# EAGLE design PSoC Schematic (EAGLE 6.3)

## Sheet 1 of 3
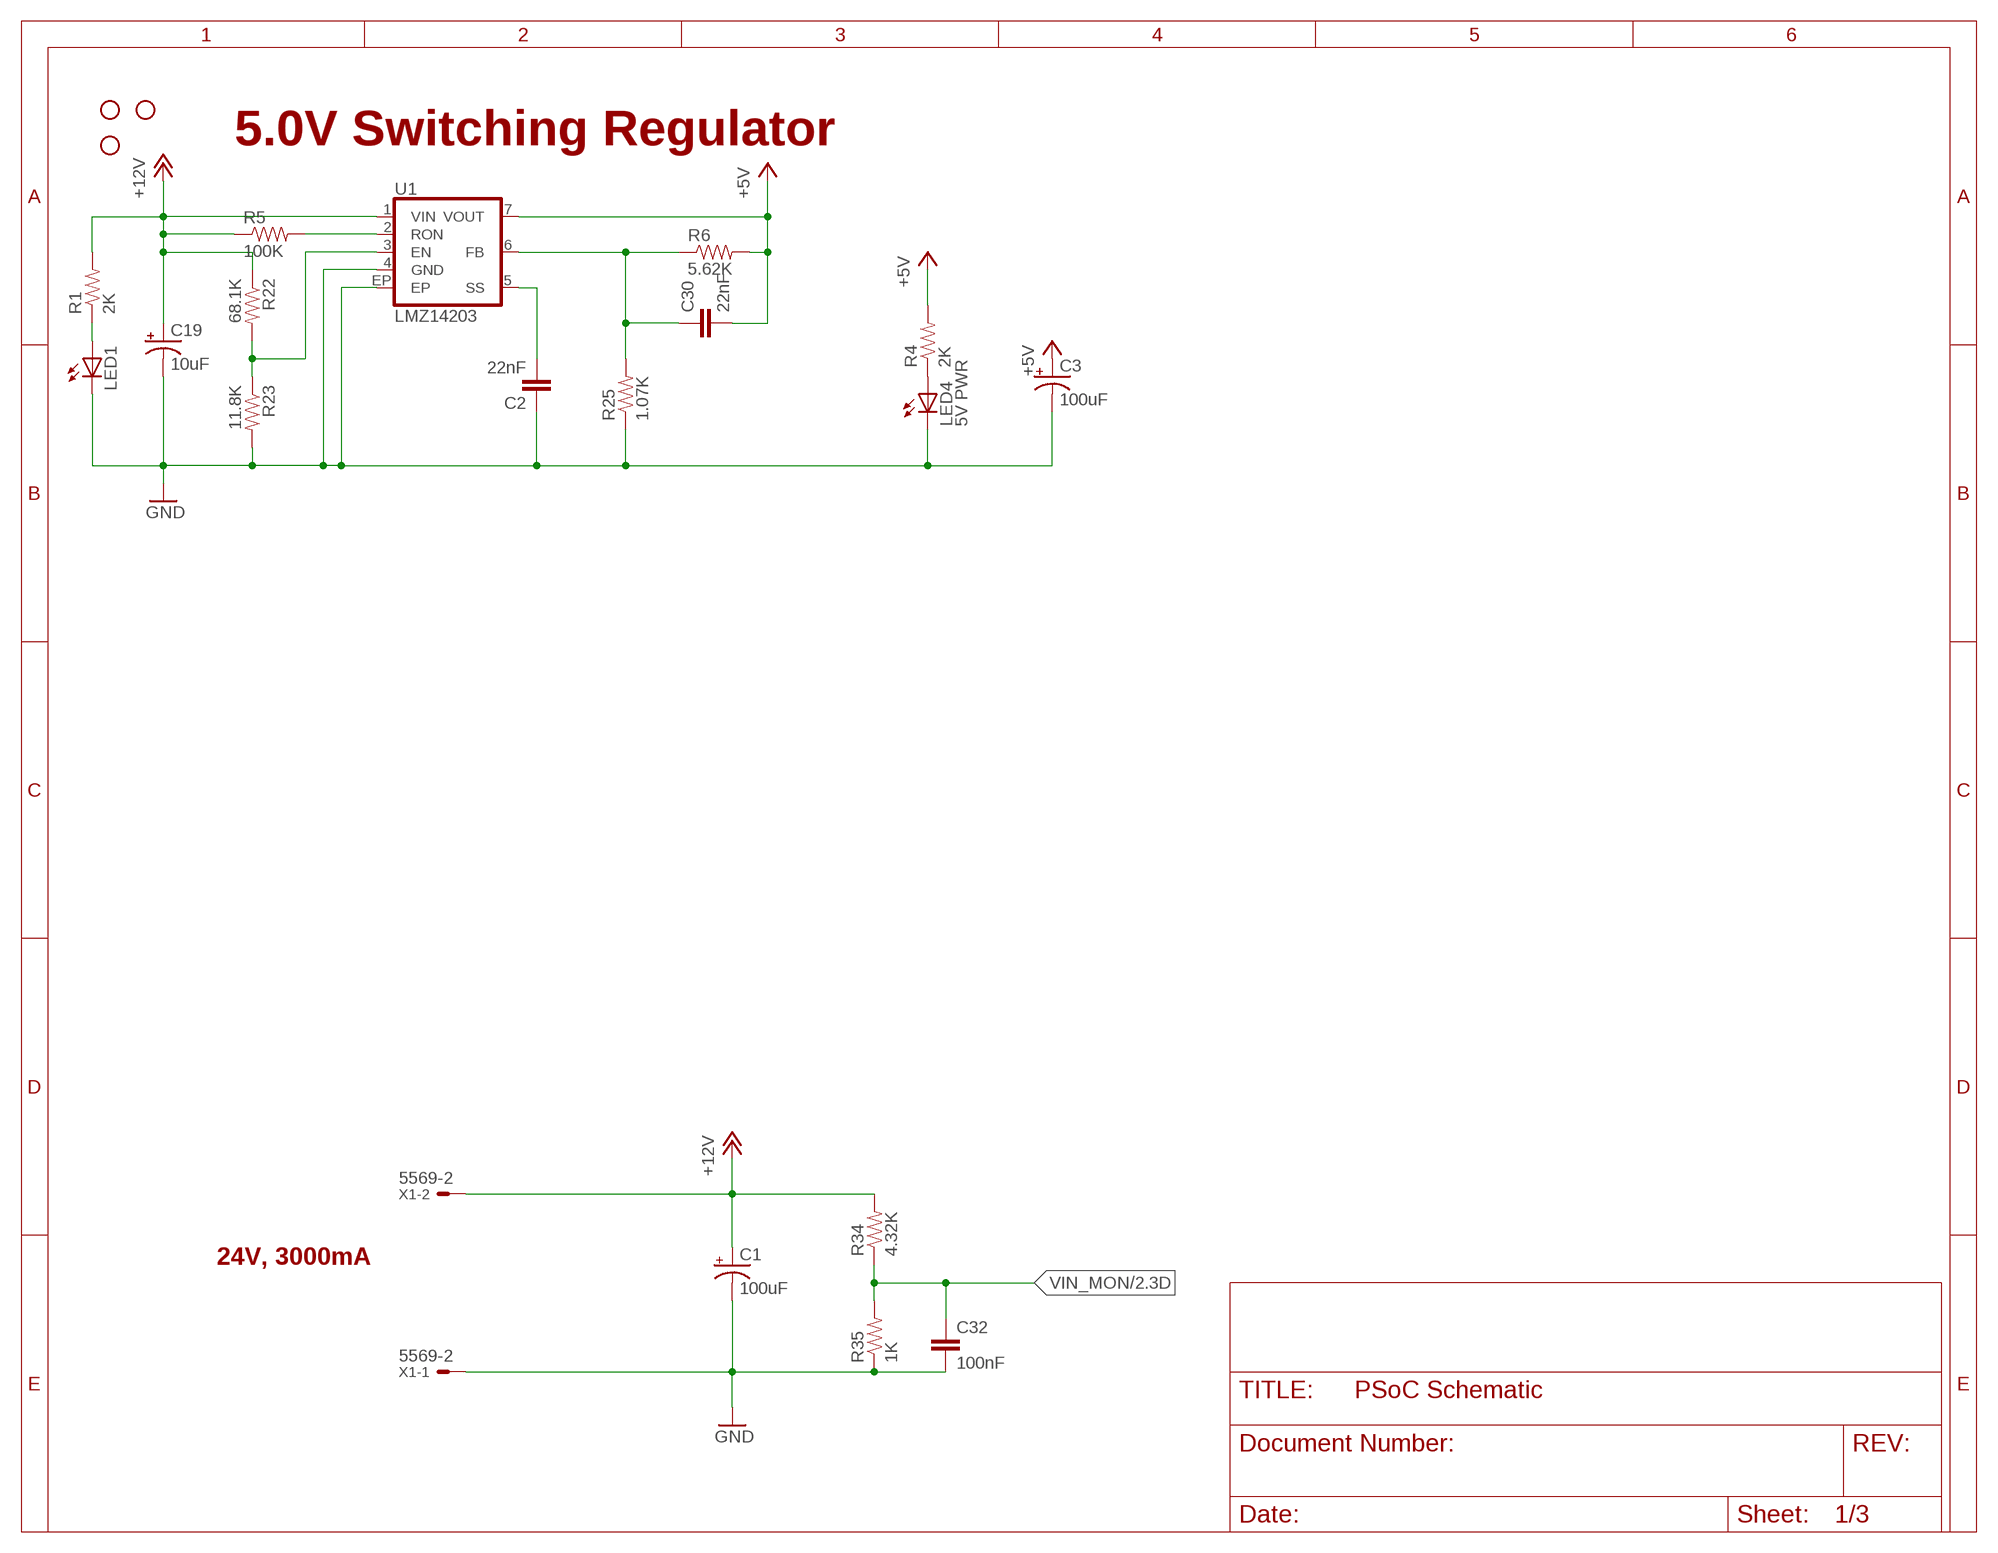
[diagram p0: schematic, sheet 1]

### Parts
C1  100uF  CAP_POLE  [PANASONIC_E]
C2  22nF  22UF-6.3V-20%(0805)  [0805]
C3  100uF  CAP_POLE  [PANASONIC_E]
C19  10uF  CAP_POL3528  [EIA3528]
C30  22nF  CAP1206  [1206]
C32  100nF  CAP1206  [1206]
JP6  SPARKFUN_STAND-OFF  [SPARKFUN_STAND-OFF]
JP7  SPARKFUN_STAND-OFF  [SPARKFUN_STAND-OFF]
JP8  SPARKFUN_STAND-OFF  [SPARKFUN_STAND-OFF]
LED1  LED1206  [LED-1206]
LED4  5V PWR  LED1206  [LED-1206]
R1  2K  RESISTOR1206  [1206]
R4  2K  RESISTOR1206  [1206]
R5  100K  RESISTOR0805-RES  [0805]
R6  5.62K  RESISTOR0805-RES  [0805]
R22  68.1K  RESISTOR1206  [1206]
R23  11.8K  RESISTOR1206  [1206]
R25  1.07K  RESISTOR1206  [1206]
R34  4.32K  RESISTOR1206  [1206]
R35  1K  RESISTOR1206  [1206]
U1  LMZ14203  [TO-PMOD-7]
U$2  MUD  [MUD]
X1  5569-2  [5569-2]

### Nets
+5V: C3.+ C30.2 R4.2 R6.2 U1.7(VOUT) ; also sheet 2,3
+12V: C1.+ C19.A(+) R1.2 R5.1 R22.1 R34.2 U1.1(VIN) X1.2 ; also sheet 3
GND: C1.- C2.1 C3.- C19.C(-) C32.2 LED1.C LED4.C R23.2 R25.1 R35.1 U1.4(GND) U1.EP X1.1 ; also sheet 2,3
N$2: LED4.A R4.1
N$3: LED1.A R1.1
N$60: R5.2 U1.2(RON)
N$62: R22.2 R23.1 U1.3(EN)
N$66: C2.2 U1.5(SS)
N$67: C30.1 R6.1 R25.2 U1.6(FB)
VIN_MON: C32.1 R34.1 R35.2 ; also sheet 2

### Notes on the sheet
- 5.0V Switching Regulator
- 24V, 3000mA

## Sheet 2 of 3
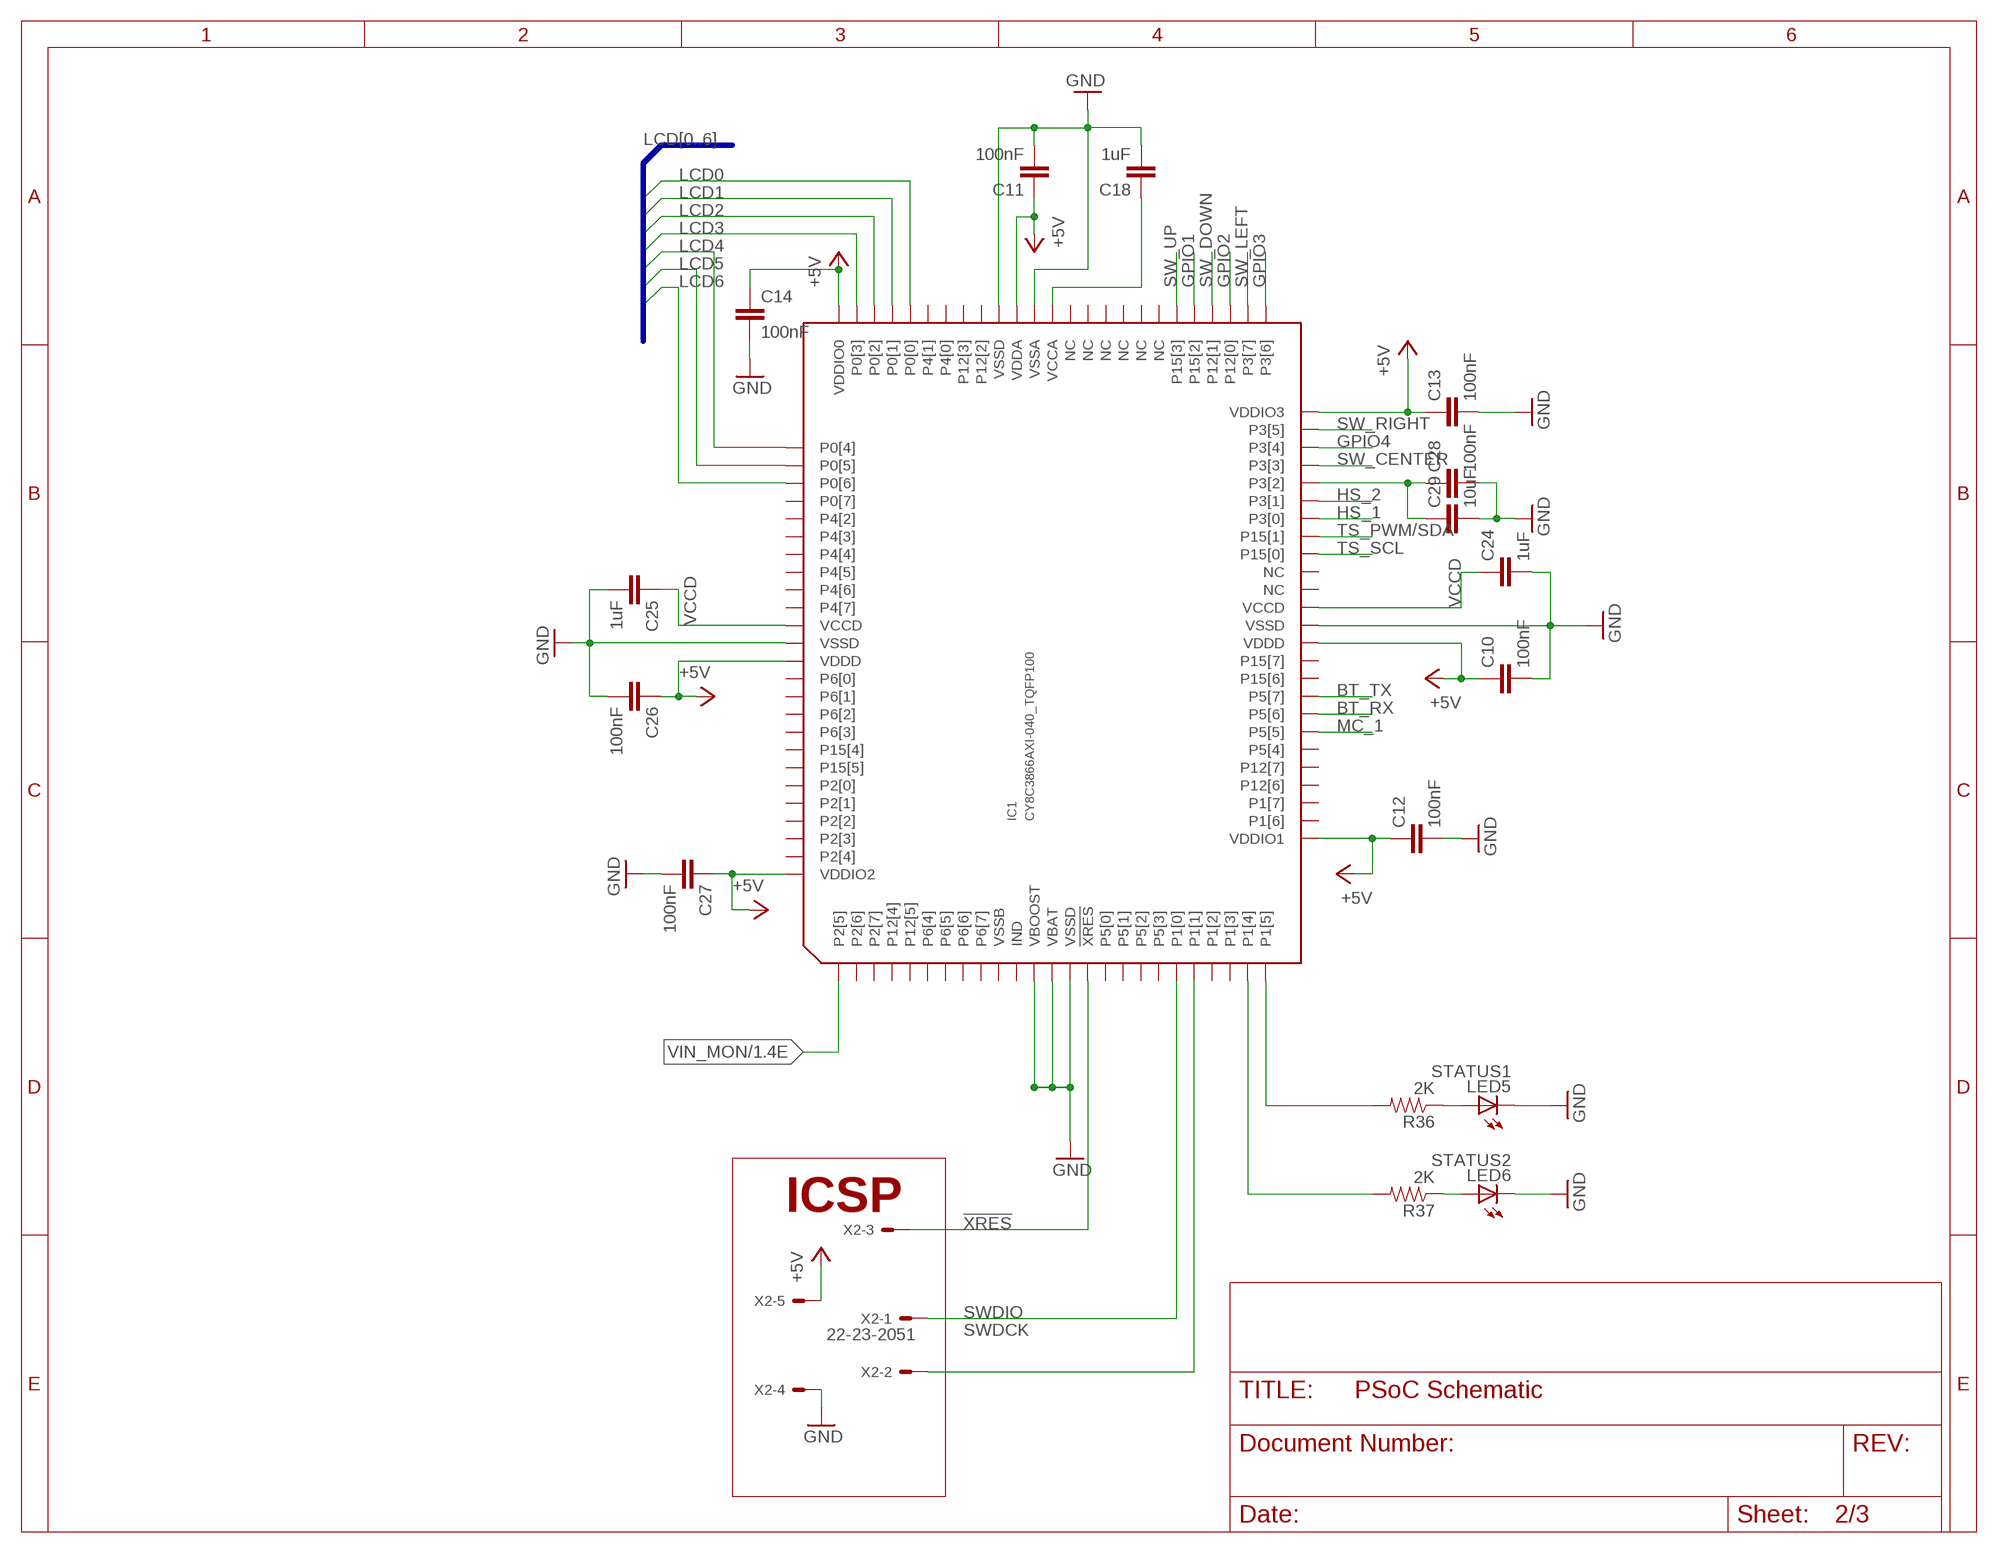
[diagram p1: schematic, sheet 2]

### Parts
C10  100nF  CAP1206  [1206]
C11  100nF  CAP1206  [1206]
C12  100nF  CAP1206  [1206]
C13  100nF  CAP1206  [1206]
C14  100nF  CAP1206  [1206]
C18  1uF  CAP1206  [1206]
C24  1uF  CAP1206  [1206]
C25  1uF  CAP1206  [1206]
C26  100nF  CAP1206  [1206]
C27  100nF  CAP1206  [1206]
C28  100nF  CAP1206  [1206]
C29  10uF  CAP1206  [1206]
IC1  CY8C3866AXI-040_TQFP100  [TQFP100]
LED5  STATUS1  LED1206  [LED-1206]
LED6  STATUS2  LED1206  [LED-1206]
R36  2K  RESISTOR1206  [1206]
R37  2K  RESISTOR1206  [1206]
X2  22-23-2051  [22-23-2051]

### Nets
!XRES: IC1.15(!XRES) X2.3
+5V: C10.1 C11.1 C12.1 C13.1 C14.1 C26.1 C27.1 IC1.26(VDDIO1) IC1.37(VDDD) IC1.50(VDDIO3) IC1.65(VDDA) IC1.75(VDDIO0) IC1.88(VDDD) IC1.100(VDDIO2) X2.5 ; also sheet 1,3
BT_RX: IC1.33(P5[6]) ; also sheet 3
BT_TX: IC1.34(P5[7]) ; also sheet 3
GND: C10.2 C11.2 C12.2 C13.2 C14.2 C18.2 C24.2 C25.2 C26.2 C27.2 C28.2 C29.2 IC1.12(VBOOST) IC1.13(VBAT) IC1.14(VSSD) IC1.38(VSSD) IC1.64(VSSA) IC1.66(VSSD) IC1.87(VSSD) LED5.C LED6.C X2.4 ; also sheet 1,3
GPIO1: IC1.55(P15[2]) ; also sheet 3
GPIO2: IC1.53(P12[0]) ; also sheet 3
GPIO3: IC1.51(P3[6]) ; also sheet 3
GPIO4: IC1.48(P3[4]) ; also sheet 3
HS_1: IC1.44(P3[0]) ; also sheet 3
HS_2: IC1.45(P3[1]) ; also sheet 3
LCD0: IC1.71(P0[0]) ; also sheet 3
LCD1: IC1.72(P0[1]) ; also sheet 3
LCD2: IC1.73(P0[2]) ; also sheet 3
LCD3: IC1.74(P0[3]) ; also sheet 3
LCD4: IC1.76(P0[4]) ; also sheet 3
LCD5: IC1.77(P0[5]) ; also sheet 3
LCD6: IC1.78(P0[6]) ; also sheet 3
MC_1: IC1.32(P5[5]) ; also sheet 3
N$10: LED5.A R36.1
N$20: IC1.25(P1[5]) R36.2
N$26: C18.1 IC1.63(VCCA)
N$28: C28.1 C29.1 IC1.46(P3[2])
N$29: LED6.A R37.1
N$32: IC1.24(P1[4]) R37.2
SW_CENTER: IC1.47(P3[3]) ; also sheet 3
SW_DOWN: IC1.54(P12[1]) ; also sheet 3
SW_LEFT: IC1.52(P3[7]) ; also sheet 3
SW_RIGHT: IC1.49(P3[5]) ; also sheet 3
SW_UP: IC1.56(P15[3]) ; also sheet 3
SWDCK: IC1.21(P1[1]) X2.2
SWDIO: IC1.20(P1[0]) X2.1
TS_PWM/SDA: IC1.43(P15[1]) ; also sheet 3
TS_SCL: IC1.42(P15[0]) ; also sheet 3
VCCD: C24.1 C25.1 IC1.39(VCCD) IC1.86(VCCD)
VIN_MON: IC1.1(P2[5]) ; also sheet 1
Unconnected: IC1.2(P2[6]) IC1.3(P2[7]) IC1.4(P12[4]) IC1.5(P12[5]) IC1.6(P6[4]) IC1.7(P6[5]) IC1.8(P6[6]) IC1.9(P6[7]) IC1.11(IND) IC1.16(P5[0]) IC1.17(P5[1]) IC1.18(P5[2]) IC1.19(P5[3]) IC1.22(P1[2]) IC1.23(P1[3]) IC1.27(P1[6]) IC1.28(P1[7]) IC1.29(P12[6]) IC1.30(P12[7]) IC1.31(P5[4]) IC1.35(P15[6]) IC1.36(P15[7]) IC1.40(NC) IC1.41(NC) IC1.57(NC) IC1.58(NC) IC1.59(NC) IC1.60(NC) IC1.61(NC) IC1.62(NC) IC1.67(P12[2]) IC1.68(P12[3]) IC1.69(P4[0]) IC1.70(P4[1]) IC1.79(P0[7]) IC1.80(P4[2]) IC1.81(P4[3]) IC1.82(P4[4]) IC1.83(P4[5]) IC1.84(P4[6]) IC1.85(P4[7]) IC1.89(P6[0]) IC1.90(P6[1]) IC1.91(P6[2]) IC1.92(P6[3]) IC1.93(P15[4]) IC1.94(P15[5]) IC1.95(P2[0]) IC1.96(P2[1]) IC1.97(P2[2]) IC1.98(P2[3]) IC1.99(P2[4])

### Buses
LCD[0..6]

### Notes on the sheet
- ICSP

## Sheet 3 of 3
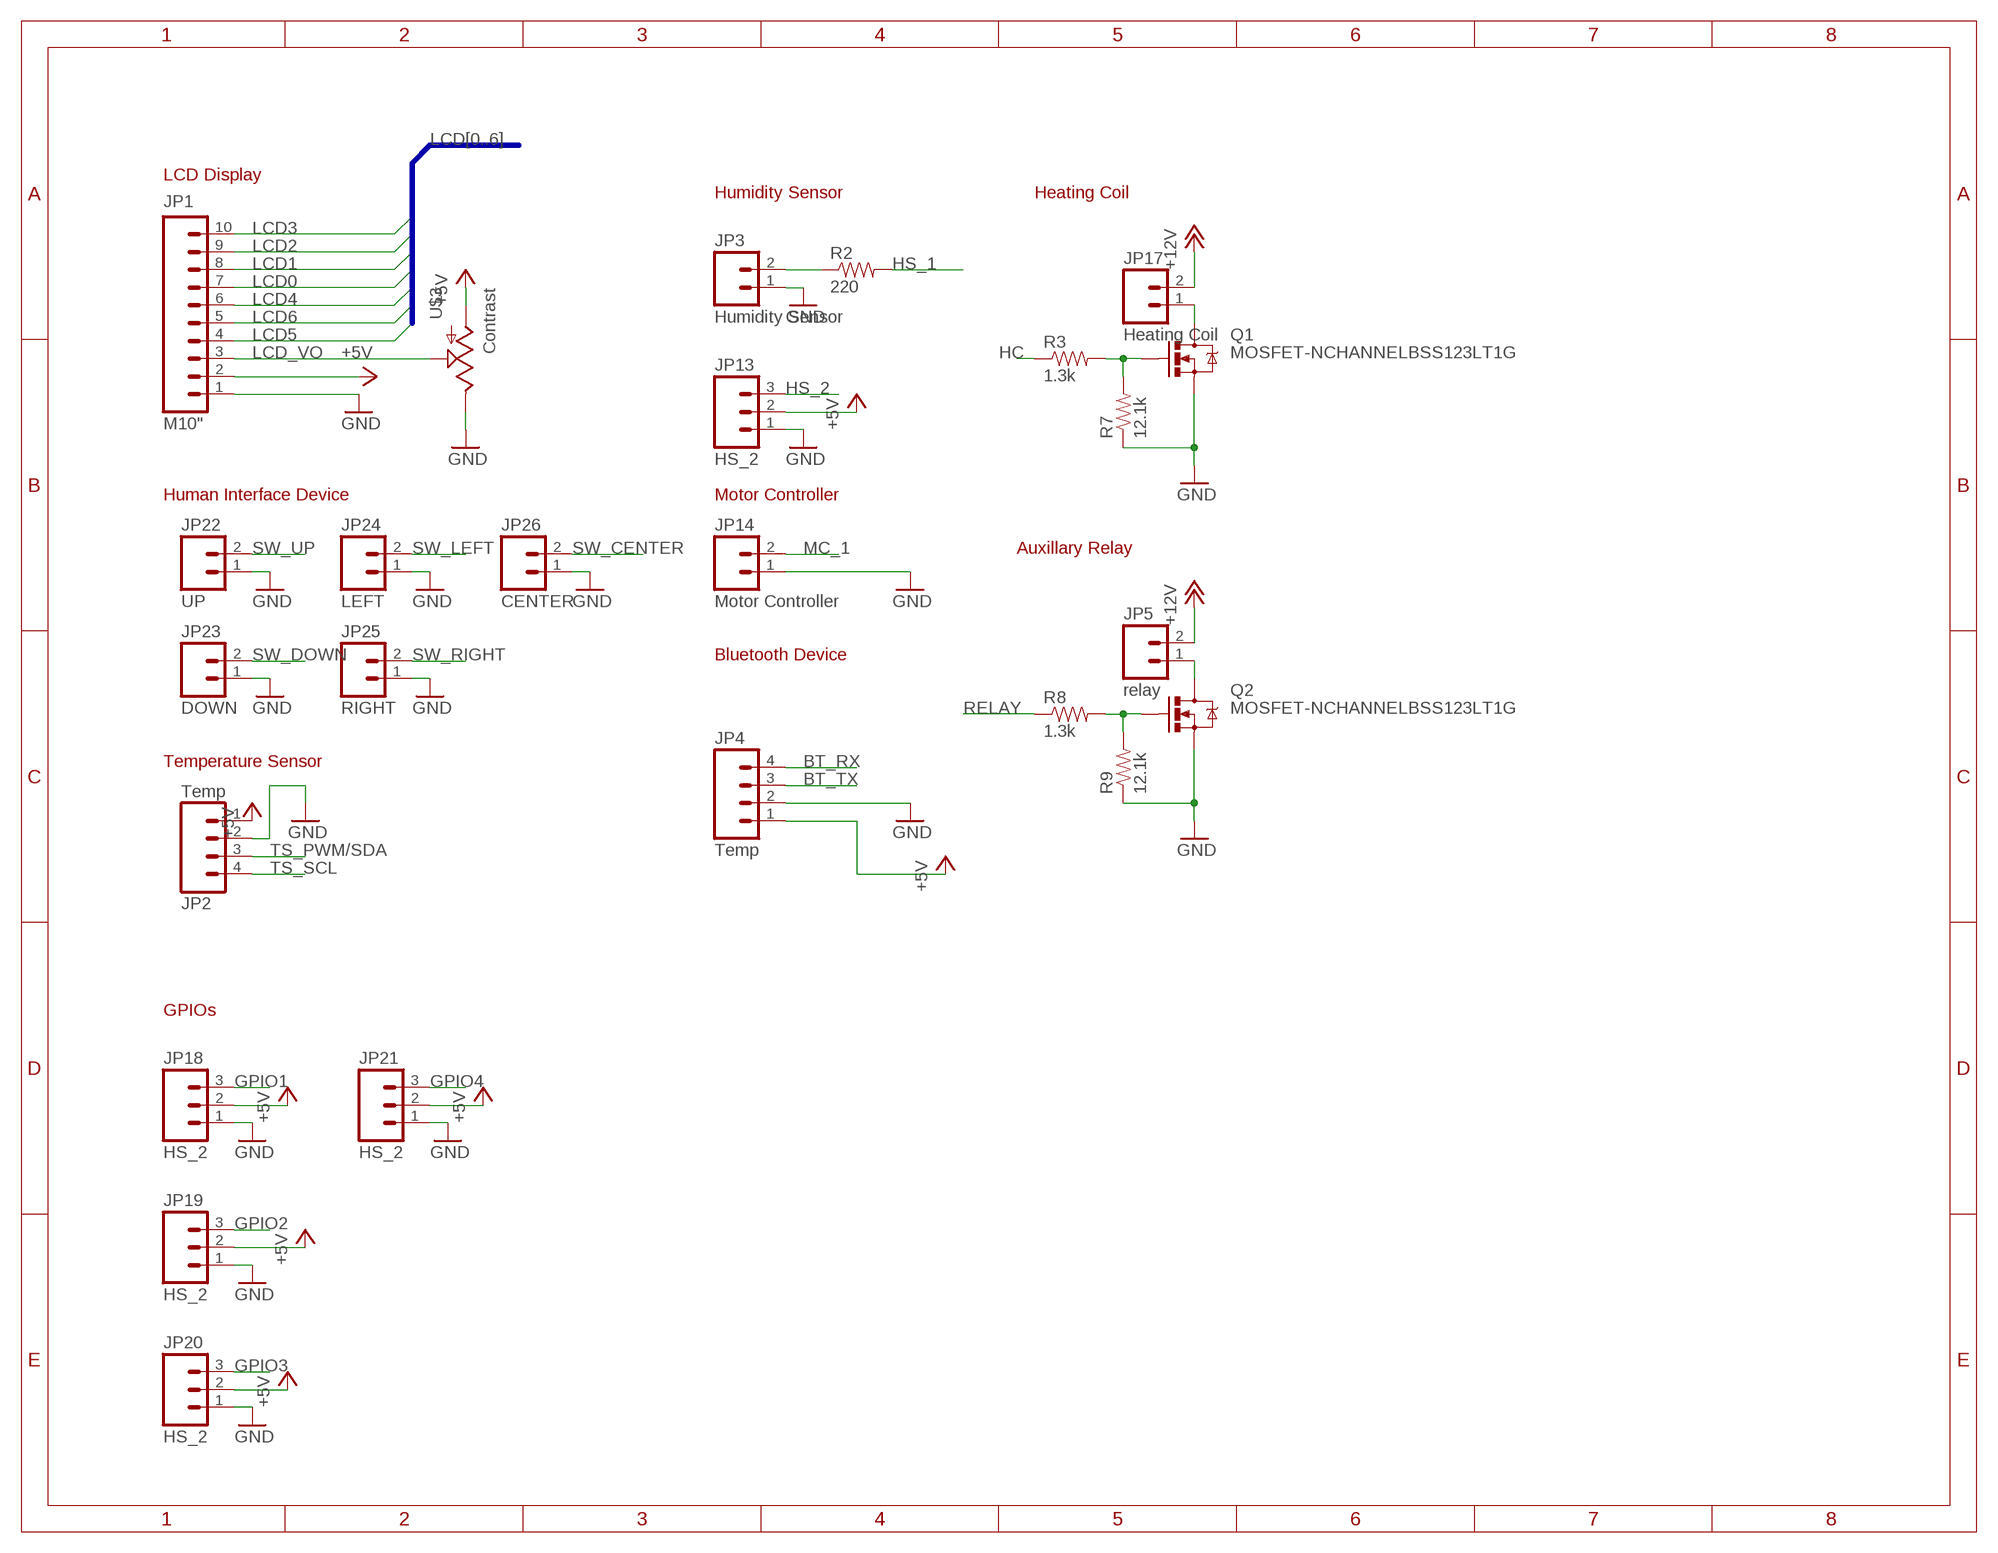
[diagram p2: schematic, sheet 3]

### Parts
JP1  M10"  [1X10]
JP2  Temp  M04POLAR  [MOLEX-1X4]
JP3  Humidity Sensor  M02POLAR  [MOLEX-1X2]
JP4  Temp  M04POLAR  [MOLEX-1X4]
JP5  relay  M02POLAR  [MOLEX-1X2]
JP13  HS_2  M03POLAR  [MOLEX-1X3]
JP14  Motor Controller  M02POLAR  [MOLEX-1X2]
JP17  Heating Coil  M02POLAR  [MOLEX-1X2]
JP18  HS_2  M03POLAR  [MOLEX-1X3]
JP19  HS_2  M03POLAR  [MOLEX-1X3]
JP20  HS_2  M03POLAR  [MOLEX-1X3]
JP21  HS_2  M03POLAR  [MOLEX-1X3]
JP22  UP  M02POLAR  [MOLEX-1X2]
JP23  DOWN  M02POLAR  [MOLEX-1X2]
JP24  LEFT  M02POLAR  [MOLEX-1X2]
JP25  RIGHT  M02POLAR  [MOLEX-1X2]
JP26  CENTER  M02POLAR  [MOLEX-1X2]
Q1  MOSFET-NCHANNELBSS123LT1G  [SOT23]
Q2  MOSFET-NCHANNELBSS123LT1G  [SOT23]
R2  220  220-5%  [0603-RES]
R3  1.3k  RESISTOR1206  [1206]
R7  12.1k  RESISTOR1206  [1206]
R8  1.3k  RESISTOR1206  [1206]
R9  12.1k  RESISTOR1206  [1206]
U$3  Contrast  POT100K_3362U  [3362U]

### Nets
+5V: JP1.2 JP2.1 JP4.1 JP13.2 JP18.2 JP19.2 JP20.2 JP21.2 U$3.P$3(A) ; also sheet 1,2
+12V: JP5.2 JP17.2 ; also sheet 1
BT_RX: JP4.4 ; also sheet 2
BT_TX: JP4.3 ; also sheet 2
GND: JP1.1 JP2.2 JP3.1 JP4.2 JP13.1 JP14.1 JP18.1 JP19.1 JP20.1 JP21.1 JP22.1 JP23.1 JP24.1 JP25.1 JP26.1 Q1.2(S) Q2.2(S) R7.1 R9.1 U$3.P$1(E) ; also sheet 1,2
GPIO1: JP18.3 ; also sheet 2
GPIO2: JP19.3 ; also sheet 2
GPIO3: JP20.3 ; also sheet 2
GPIO4: JP21.3 ; also sheet 2
HC: R3.1
HS_1: R2.2 ; also sheet 2
HS_2: JP13.3 ; also sheet 2
LCD0: JP1.7 ; also sheet 2
LCD1: JP1.8 ; also sheet 2
LCD2: JP1.9 ; also sheet 2
LCD3: JP1.10 ; also sheet 2
LCD4: JP1.6 ; also sheet 2
LCD5: JP1.4 ; also sheet 2
LCD6: JP1.5 ; also sheet 2
LCD_VO: JP1.3 U$3.P$2(S)
MC_1: JP14.2 ; also sheet 2
N$1: JP3.2 R2.1
N$4: Q1.1(G) R3.2 R7.2
N$5: JP17.1 Q1.3(D)
N$7: Q2.1(G) R8.2 R9.2
N$8: JP5.1 Q2.3(D)
RELAY: R8.1
SW_CENTER: JP26.2 ; also sheet 2
SW_DOWN: JP23.2 ; also sheet 2
SW_LEFT: JP24.2 ; also sheet 2
SW_RIGHT: JP25.2 ; also sheet 2
SW_UP: JP22.2 ; also sheet 2
TS_PWM/SDA: JP2.3 ; also sheet 2
TS_SCL: JP2.4 ; also sheet 2

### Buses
LCD[0..6]

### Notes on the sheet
- LCD Display
- Humidity Sensor | Heating Coil
- Human Interface Device | Motor Controller
- Auxillary Relay
- Bluetooth Device
- Temperature Sensor
- GPIOs

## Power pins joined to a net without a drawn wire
VSSB: IC1.10(VSSB)

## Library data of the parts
C1 C3 C19 = SparkFun:CAP_POL: Capacitor Polarized
C2 = SparkFun-Capacitors:22UF-6.3V-20%(0805): Ceramic; PROD_ID: CAP-08402; VALUE: 22uF
C10-C14 C18 C24-C30 C32 = SparkFun:CAP: Capacitor
IC1 = cypresspsoc_0.30:CY8C3866AXI-040
JP1 = SparkFun-Connectors:M10: Header 10 Standard 10-pin 0.1" header. Use with straight break away headers (SKU : PRT-00116), right angle break away headers (PRT-00553), swiss pins (PRT-00743), machine pins (PRT-00117), and female headers (PRT-00115).
JP2 JP4 = SparkFun-Connectors:M04: Header 4 Standard 4-pin 0.1" header. Use with straight break away headers (SKU : PRT-00116), right angle break away headers (PRT-00553), swiss pins (PRT-00743), machine pins (PRT-00117), and female headers (PRT-00115). Molex polarized connector foot print use with SKU : PRT-08231 with associated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
JP3 JP5 JP14 JP17 JP22-JP26 = SparkFun-Connectors:M02: Header 2
JP6-JP8 = IOIO-OTG-v20brandon2-14-13:SPARKFUN_STAND-OFF: Stand Off
JP13 JP18-JP21 = SparkFun-Connectors:M03: Header 3 Standard 3-pin 0.1" header. Use with straight break away headers (SKU : PRT-00116), right angle break away headers (PRT-00553), swiss pins (PRT-00743), machine pins (PRT-00117), and female headers (PRT-00115). Molex polarized connector foot print use with SKU : PRT-08232 with associated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
LED1 LED4-LED6 = SparkFun:LED: LEDs
Q1 Q2 = SparkFun-DiscreteSemi:MOSFET-NCHANNEL: Common NMOSFET Parts MFG P/NStore IDProd ID FDD8780TRANS-09984 SI7820DNTRANS-11055 FDS6630AIC-08089 2N7002PWTRANS-11151 FQP30N06L COM-10213TRANS-10060 BSS123LT1GTRANS-08345 BSS138TRANS-00830 BS170 2N7000; PROD_ID: TRANS-08345
R1 R4 R22 R23 R25 R34-R37 = SparkFun:RESISTOR: Resistor
R2 = SparkFun-Resistors:220-5%: 220-ohm SMT; PROD_ID: RES-07866
R3 R5-R9 = SparkFun-Passives:RESISTOR: Resistor
U1 = SparkFun:LMZ14203: LMZ14203 3A, Simple Switcher Power Module with 42V Maximum Input
U$2 = logo:MUD
U$3 = SparkFun-Electromechanical:POT
X1 = molex:5569-2: Mini FIT connector 2 pol; OC_FARNELL: 1822072; OC_NEWARK: unknown
X2 = con-molex:22-23-2051: .100" (2.54mm) Center Header - 5 Pin; MF: MOLEX; MPN: 22-23-2051; OC_FARNELL: 1462952; OC_NEWARK: 38C9178

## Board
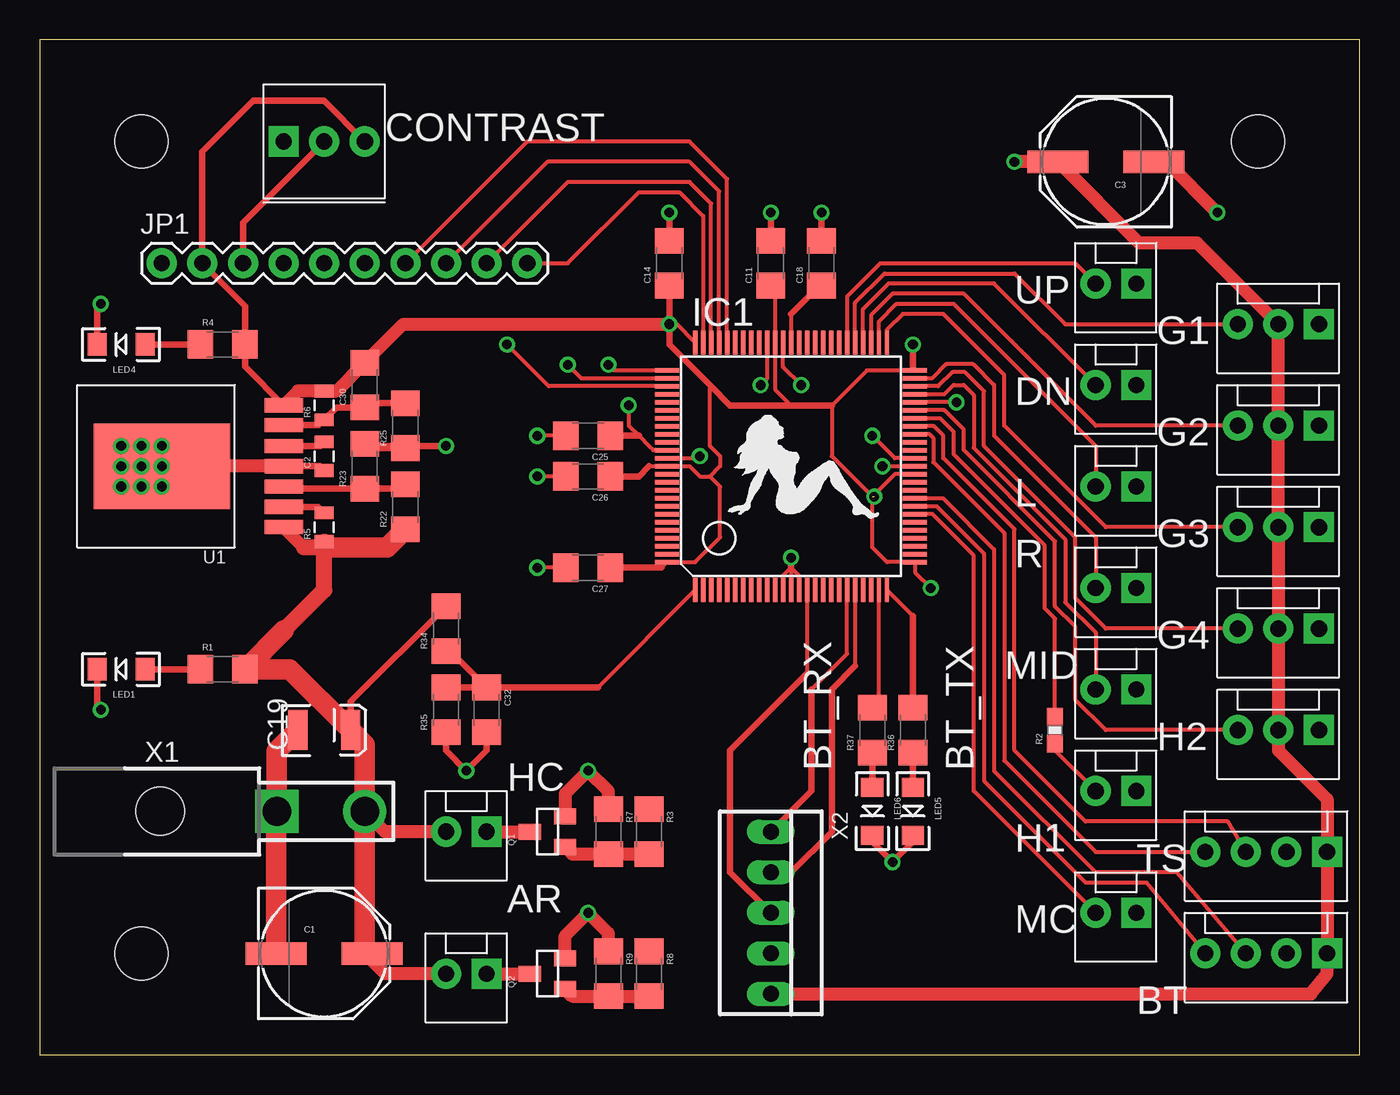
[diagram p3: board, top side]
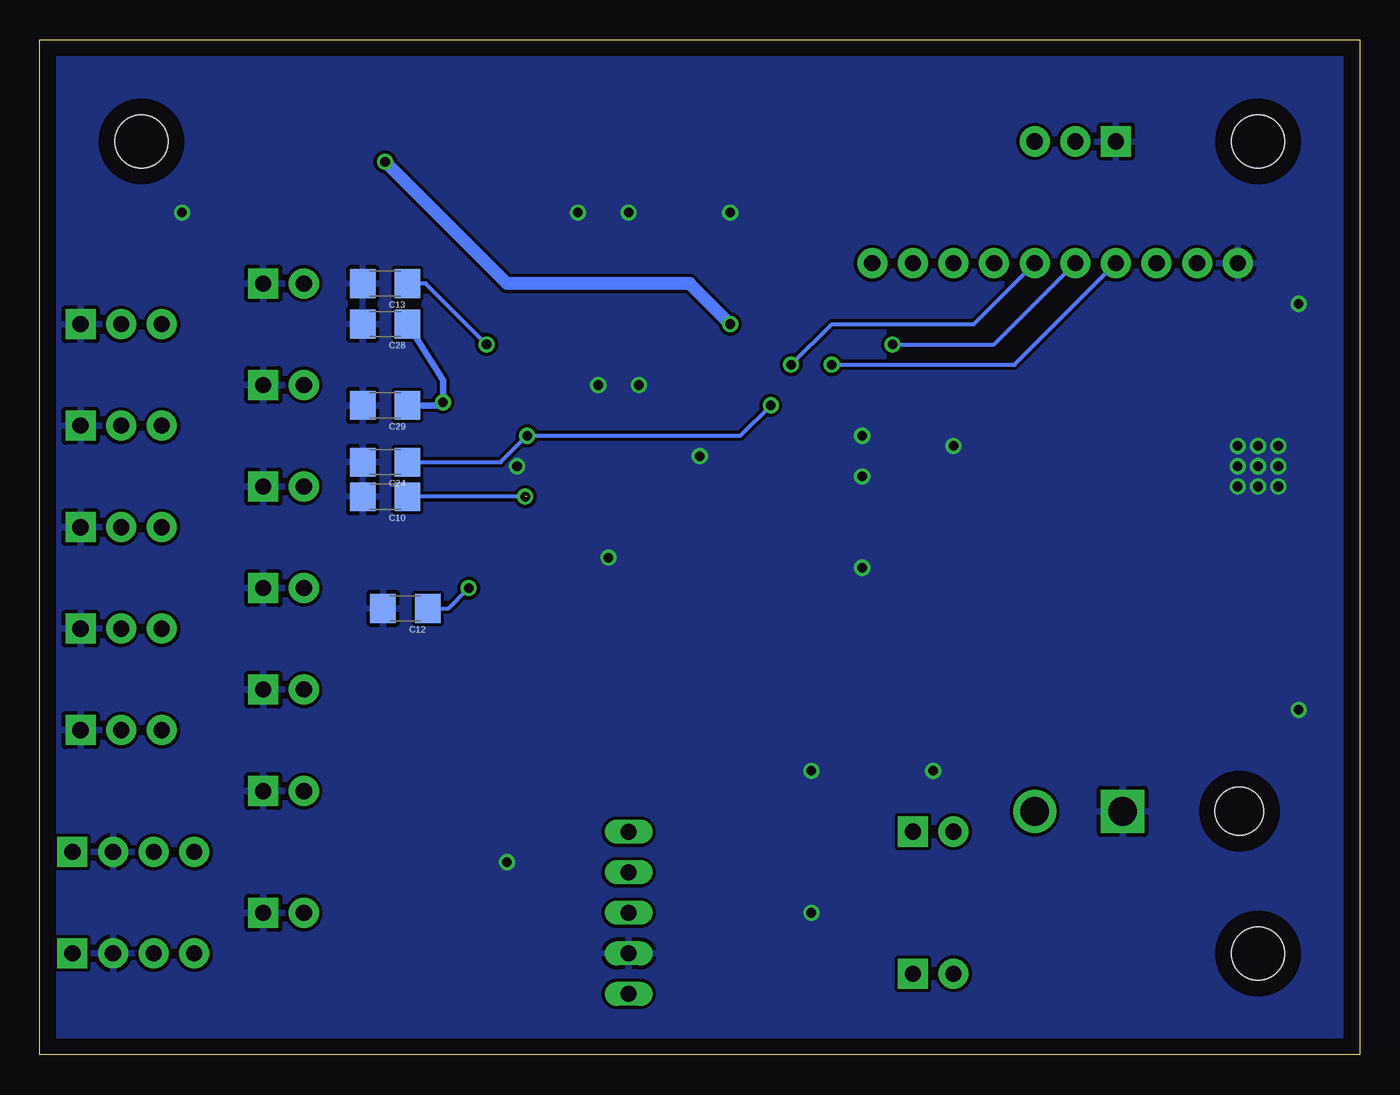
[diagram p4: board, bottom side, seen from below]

Size 82.55 x 63.5 mm. Coordinates in mm from the lower left corner, seen from the top.
Outline: 0,0 82.55,0 82.55,63.5 0,63.5 0,0
Copper layers (1*16): Top 0.035mm / dielectric 1.5mm / Bottom 0.035mm
Design rules "default": minimum track width 10mil, minimum drill 24mil, track to track 8mil, track to pad 8mil, pad to pad 8mil, via to via 8mil, smd to smd 8mil, copper to edge 40mil, drill to drill 8mil, minimum pad ring 10mil, minimum via ring 8mil, stop-mask expansion 4mil, vias tented up to drill 0mil, thermal gap 10mil

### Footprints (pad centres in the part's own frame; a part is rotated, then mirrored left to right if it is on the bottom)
PANASONIC_E = smd 3.8 x 1.4: + 3,0; - -3,0
0805 = smd 0.8 x 1.2: 1 -0.9,0; 2 0.9,0
1206 = smd 1.6 x 1.8: 1 -1.4,0; 2 1.4,0
EIA3528 = smd 1.2 x 2.5: A 1.65,0; C -1.65,0
TQFP100 = smd 0.27 x 1.5: 1 -6,-7.75; 2 -5.5,-7.75; 3 -5,-7.75; 4 -4.5,-7.75; 5 -4,-7.75; 6 -3.5,-7.75; 7 -3,-7.75; 8 -2.5,-7.75; 9 -2,-7.75; 10 -1.5,-7.75; 11 -1,-7.75; 12 -0.5,-7.75; 13 0,-7.75; 14 0.5,-7.75; 15 1,-7.75; 16 1.5,-7.75; 17 2,-7.75; 18 2.5,-7.75; 19 3,-7.75; 20 3.5,-7.75; 21 4,-7.75; 22 4.5,-7.75; 23 5,-7.75; 24 5.5,-7.75; 25 6,-7.75; 51 6,7.75; 52 5.5,7.75; 53 5,7.75; 54 4.5,7.75; 55 4,7.75; 56 3.5,7.75; 57 3,7.75; 58 2.5,7.75; 59 2,7.75; 60 1.5,7.75; 61 1,7.75; 62 0.5,7.75; 63 0,7.75; 64 -0.5,7.75; 65 -1,7.75; 66 -1.5,7.75; 67 -2,7.75; 68 -2.5,7.75; 69 -3,7.75; 70 -3.5,7.75; 71 -4,7.75; 72 -4.5,7.75; 73 -5,7.75; 74 -5.5,7.75; 75 -6,7.75 | smd 1.5 x 0.27: 26 7.75,-6; 27 7.75,-5.5; 28 7.75,-5; 29 7.75,-4.5; 30 7.75,-4; 31 7.75,-3.5; 32 7.75,-3; 33 7.75,-2.5; 34 7.75,-2; 35 7.75,-1.5; 36 7.75,-1; 37 7.75,-0.5; 38 7.75,0; 39 7.75,0.5; 40 7.75,1; 41 7.75,1.5; 42 7.75,2; 43 7.75,2.5; 44 7.75,3; 45 7.75,3.5; 46 7.75,4; 47 7.75,4.5; 48 7.75,5; 49 7.75,5.5; 50 7.75,6; 76 -7.75,6; 77 -7.75,5.5; 78 -7.75,5; 79 -7.75,4.5; 80 -7.75,4; 81 -7.75,3.5; 82 -7.75,3; 83 -7.75,2.5; 84 -7.75,2; 85 -7.75,1.5; 86 -7.75,1; 87 -7.75,0.5; 88 -7.75,0; 89 -7.75,-0.5; 90 -7.75,-1; 91 -7.75,-1.5; 92 -7.75,-2; 93 -7.75,-2.5; 94 -7.75,-3; 95 -7.75,-3.5; 96 -7.75,-4; 97 -7.75,-4.5; 98 -7.75,-5; 99 -7.75,-5.5; 100 -7.75,-6
1X10 = drill 1.016 pad 1.88: 1 0,0; 2 2.54,0; 3 5.08,0; 4 7.62,0; 5 10.16,0; 6 12.7,0; 7 15.24,0; 8 17.78,0; 9 20.32,0; 10 22.86,0
MOLEX-1X4 = drill 1.016 pad 1.88 square: 1 0,0 | drill 1.016 pad 1.88: 2 2.54,0; 3 5.08,0; 4 7.62,0
MOLEX-1X2 = drill 1.016 pad 1.88 square: 1 0,0 | drill 1.016 pad 1.88: 2 2.54,0
SPARKFUN_STAND-OFF = hole 3.302: 0,0
MOLEX-1X3 = drill 1.016 pad 1.88 square: 1 0,0 | drill 1.016 pad 1.88: 2 2.54,0; 3 5.08,0
LED-1206 = smd 1.2 x 1.4: A -1.5,0; C 1.5,0
SOT23 = smd 1 x 1.4: 1 -0.95,-1.1; 2 0.95,-1.1; 3 0,1.1
0603-RES = smd 1.1 x 1: 1 -0.85,0; 2 0.85,0
TO-PMOD-7 = smd 0.89 x 2.41: 1 -3.81,-7.63; 2 -2.54,-7.63; 3 -1.27,-7.63; 4 0,-7.63; 5 1.27,-7.63; 6 2.57,-7.63; 7 3.81,-7.63 | smd 5.35 x 8.54: EP 0,0
3362U = drill 1.016 pad 1.88 square: P$1 0,2.54 | drill 1.016 pad 1.88: P$2 2.54,2.54; P$3 5.08,2.54
5569-2 = drill 1.8 square: 1 0,-5.5 | drill 1.8: 2 0,0 | hole 3: 0,-12.8
22-23-2051 = drill 1 long: 1 -5.08,0; 2 -2.54,0; 3 0,0; 4 2.54,0; 5 5.08,0

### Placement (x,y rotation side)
C1  17.78,6.35 0 top
C2  17.78,37.47 90 top
C3  66.67,55.88 180 top
C10  60.96,34.92 180 bottom
C11  45.72,49.53 90 top
C12  59.69,27.94 180 bottom
C13  60.96,48.26 180 bottom
C14  39.37,49.53 90 top
C18  48.9,49.53 90 top
C19  17.78,20.32 0 top
C24  60.96,37.08 180 bottom
C25  34.29,38.73 180 top
C26  34.29,36.2 180 top
C27  34.29,30.48 180 top
C28  60.96,45.72 180 bottom
C29  60.96,40.64 180 bottom
C30  20.32,41.91 90 top
C32  27.94,21.59 270 top
IC1  46.99,36.83 0 top
JP1  7.62,49.53 0 top
JP2  80.52,12.7 180 top
JP3  68.58,16.51 180 top
JP4  80.52,6.35 180 top
JP5  27.94,5.08 180 top
JP6  6.35,6.35 0 top
JP7  6.35,57.15 0 top
JP8  76.2,57.15 0 top
JP13  80.01,20.32 180 top
JP14  68.58,8.89 180 top
JP17  27.94,13.97 180 top
JP18  80.01,45.72 180 top
JP19  80.01,39.37 180 top
JP20  80.01,33.02 180 top
JP21  80.01,26.67 180 top
JP22  68.58,48.26 180 top
JP23  68.58,41.91 180 top
JP24  68.58,35.56 180 top
JP25  68.58,29.21 180 top
JP26  68.58,22.86 180 top
LED1  5.08,24.13 180 top
LED4  5.08,44.45 180 top
LED5  54.61,15.24 270 top
LED6  52.07,15.24 270 top
Q1  31.75,13.97 90 top
Q2  31.75,5.08 90 top
R1  11.43,24.13 0 top
R2  63.5,20.32 90 top
R3  38.1,13.97 270 top
R4  11.43,44.45 0 top
R5  17.78,33.02 90 top
R6  17.78,40.64 90 top
R7  35.56,13.97 270 top
R8  38.1,5.08 270 top
R9  35.56,5.08 270 top
R22  22.86,34.29 90 top
R23  20.32,36.83 90 top
R25  22.86,39.37 90 top
R34  25.4,26.67 90 top
R35  25.4,21.59 90 top
R36  54.61,20.32 90 top
R37  52.07,20.32 90 top
U1  7.62,36.83 90 top
U$2  42.67,33.02 0 top
U$3  15.24,54.61 0 top
X1  20.32,15.24 270 top
X2  45.72,8.89 270 top

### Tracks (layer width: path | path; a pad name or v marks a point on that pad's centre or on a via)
!XRES
  Top 0.254: IC1.15 47.99,23.86
  Top 0.406: 47.99,23.86 43.18,19.05 43.18,11.43 X2.3
+5V  (via drill 0.6)  (1 unrouted)
  Top 0.254: 45.99,48.13 IC1.65 45.99,41.64 46.99,40.64 | 38.1,36.83 IC1.88 40.64,36.83 41.27,36.2 41.91,36.2 | 38.89,30.48 IC1.100 40.99,30.83 42.55,32.38 42.55,35.56 41.91,36.2 | 54.61,42.96 IC1.50 51.72,42.83 49.53,40.64 | 49.53,40.64 46.99,40.64 | 52.07,34.92 52.07,31.75 52.99,30.83 IC1.26 54.74,30.2 v55.73,29.21 | IC1.37 53.48,36.33 52.07,34.92 | 49.53,40.64 49.53,37.47 52.07,34.92 | 44.93,40.64 46.99,40.64 | 41.91,36.2 42.55,36.83 42.55,37.47 41.91,38.1 41.91,41.91 | IC1.75 39.85,45.72 v39.37,45.72
  Top 0.406: C11.1 45.99,48.13 | C26.1 37.47,36.2 38.1,36.83 | C27.1 38.89,30.48 | v54.61,44.45 54.61,42.96 | U1.7 12.83,43.06 R4.2 12.83,46.86 JP1.2 10.16,56.52 13.34,59.69 17.78,59.69 U$3.P$3 | C14.1 v39.37,45.72 39.37,44.45 41.91,41.91 43.18,40.64 49.53,40.64
  Top 0.813: v39.37,45.72 22.73,45.72 C30.2 18.55,41.54 R6.2 16.15,41.54 U1.7 | v60.96,55.88 C3.+ 68.75,50.8 72.39,50.8 JP18.2 JP19.2 JP20.2 JP21.2 JP13.2 77.47,19.05 80.52,16 JP2.1 JP4.1 80.52,5.08 79.5,3.81 X2.5
  Bottom 0.254: v54.61,44.45 58.42,48.26 C13.1 | C12.1 56.99,27.94 v55.73,29.21 | v52.2,34.92 C10.1
  Bottom 0.813: v39.37,45.72 41.91,48.26 53.34,48.26 v60.96,55.88
+12V
  Top 0.406: R34.2 19.43,22.1 C19.A
  Top 0.813: JP5.2 21.59,5.08 20.32,6.35 C1.+ | JP17.2 21.59,13.97 X1.2 | 16.51,31.75 U1.1
  Top 1.016: 15.25,26.55 17.78,29.08 17.78,31.75 R5.1 17.41,31.75 16.51,31.75
  Top 1.27: C1.+ 20.32,6.81 X1.2 20.32,19.43 C19.A 15.62,24.13 R1.2 15.25,26.55 | R22.1 21.72,31.75 17.78,31.75
BT_RX
  Top 0.254: IC1.33 56.09,34.33 59.05,31.37 59.05,17.14 65.41,10.79 69.22,10.79 JP4.4
BT_TX
  Top 0.254: JP4.3 71.12,11.43 66.04,11.43 59.69,17.78 59.69,31.62 56.48,34.83 IC1.34
GND  (via drill 0.6)
  Top 0.254: IC1.66 45.49,42.31 v45.09,41.91 | 46.99,30.48 IC1.13 | IC1.12 46.49,29.98 46.99,30.48 | IC1.14 47.49,29.98 46.99,30.48 | v52.7,36.83 IC1.38 | v47.62,41.91 46.49,43.05 IC1.64 | IC1.87 41.14,37.33 v41.27,37.47 | C25.2 v31.11,38.73 | C26.2 v31.11,36.2 | C27.2 v31.11,30.48
  Top 0.406: C11.2 v45.72,52.7 | v48.9,52.7 C18.2 | v39.37,52.7 C14.2 39.37,50.8 | v46.99,31.11 46.99,30.48 | LED6.C 52.07,13.34 v53.34,12.06 54.61,13.34 LED5.C | C2.1 17.52,36.83 U1.4 | R25.1 20.58,37.97 R23.2 20.45,38.1 v25.4,38.1 | LED4.C 3.58,46.76 v3.81,46.99 | R35.1 25.4,19.05 v26.67,17.78 27.94,19.05 C32.2 | LED1.C 3.58,21.82 v3.81,21.59
  Top 0.813: U1.4 U1.EP | R7.1 35.56,16.51 v34.29,17.78 32.85,16.34 Q1.2 | R9.1 35.56,7.62 v34.29,8.89 32.85,7.45 Q2.2 | C3.- 70.48,55.88 v73.66,52.7
  Top 1.27: C19.C 14.82,19.01 X1.1 14.78,15.2 C1.-
  other vias: 7.62,36.83 7.62,38.1 6.35,38.1 5.08,38.1 5.08,36.83 6.35,36.83 5.08,35.56 6.35,35.56 7.62,35.56
  pour Bottom: 0,63.5 0,0 82.55,0 82.55,63.5
GPIO1
  Top 0.254: IC1.55 50.99,47.05 52.83,48.9 60.96,48.9 64.14,45.72 JP18.3
GPIO2
  Top 0.254: JP19.3 66.04,39.37 57.78,47.62 53.34,47.62 51.99,46.27 IC1.53
GPIO3
  Top 0.254: IC1.51 52.99,45.37 53.98,46.35 56.52,46.35 60.33,42.55 60.33,39.37 66.67,33.02 JP20.3
GPIO4
  Top 0.254: JP21.3 66.67,26.67 64.77,28.57 64.77,32.38 59.05,38.1 59.05,41.53 57.87,42.72 57.07,42.72 56.18,41.83 IC1.48
HS_1
  Top 0.254: IC1.44 56.31,39.83 57.15,38.99 57.15,37.59 62.87,31.88 62.87,27.94 63.5,27.3 R2.2
HS_2
  Top 0.254: JP13.3 66.67,20.32 64.77,22.23 64.77,26.8 63.5,28.07 63.5,32.13 57.78,37.85 57.78,39.12 56.57,40.33 IC1.45
LCD0
  Top 0.254: IC1.71 42.99,54.8 40.64,57.15 30.48,57.15 JP1.7
LCD1
  Top 0.254: IC1.72 42.49,54.03 40.64,55.88 31.75,55.88 JP1.8
LCD2
  Top 0.254: IC1.73 41.99,53.26 40.64,54.61 33.02,54.61 JP1.9
LCD3
  Top 0.254: JP1.10 33.02,49.53 37.47,53.98 40.01,53.98 41.49,52.49 IC1.74
LCD4  (via drill 0.6)
  Top 0.254: IC1.76 35.91,42.83 v35.56,43.18
  Bottom 0.254: v35.56,43.18 33.02,45.72 24.13,45.72 JP1.6
LCD5  (via drill 0.6)
  Top 0.254: IC1.77 33.87,42.33 v33.02,43.18
  Bottom 0.254: v33.02,43.18 21.59,43.18 JP1.4
LCD6  (via drill 0.6)
  Top 0.254: IC1.78 31.83,41.83 v29.21,44.45
  Bottom 0.254: v29.21,44.45 22.86,44.45 JP1.5
LCD_VO
  Top 0.406: U$3.P$2 12.7,52.07 JP1.3
MC_1
  Top 0.254: JP14.2 58.42,16.51 58.42,31.24 55.83,33.83 IC1.32
N$1
  Top 0.254: R2.1 63.5,19.05 JP3.2
N$2
  Top 0.406: LED4.A R4.1
N$3
  Top 0.406: R1.1 LED1.A
N$4
  Top 0.813: Q1.1 33.3,12.57 R7.2 R3.2
N$5
  Top 0.813: JP17.1 Q1.3
N$7
  Top 0.813: Q2.1 33.3,3.68 R9.2 R8.2
N$8
  Top 0.813: JP5.1 Q2.3
N$10
  Top 0.406: R36.1 LED5.A
N$20
  Top 0.254: IC1.25 54.61,27.46
  Top 0.406: 54.61,27.46 R36.2
N$26
  Top 0.254: 46.99,46.35 IC1.63
  Top 0.406: C18.1 48.77,48.13 46.99,46.35
N$28  (via drill 0.6)
  Top 0.254: v57.34,40.83 IC1.46
  Bottom 0.406: C29.1 57.53,40.64 v57.34,40.83 57.34,42.23 C28.1
N$29
  Top 0.406: R37.1 LED6.A
N$32
  Top 0.254: 52.49,22.14 IC1.24
  Top 0.406: R37.2 52.49,22.14
N$60
  Top 0.406: U1.2 17.41,34.29 R5.2
N$62
  Top 0.406: U1.3 15.38,35.43 R23.1 22.6,35.43 R22.2
N$66
  Top 0.406: C2.2 17.52,38.1 U1.5
N$67
  Top 0.406: U1.6 17.44,39.4 R6.1 18.55,40.51 C30.1 20.58,40.77 R25.2
SW_CENTER
  Top 0.254: IC1.47 56.57,41.33 57.15,41.91 57.78,41.91 58.42,41.27 58.42,37.97 64.14,32.26 64.14,28.32 66.04,26.42 JP26.2
SW_DOWN
  Top 0.254: JP23.2 59.69,48.26 53.09,48.26 51.49,46.66 IC1.54
SW_LEFT
  Top 0.254: IC1.52 52.49,45.89 53.59,46.99 57.15,46.99 66.04,38.1 JP24.2
SW_RIGHT
  Top 0.254: JP25.2 66.04,32.38 59.69,38.73 59.69,41.91 58.38,43.22 56.68,43.22 55.79,42.33 IC1.49
SW_UP
  Top 0.254: IC1.56 50.49,47.44 52.58,49.53 64.77,49.53 JP22.2
SWDCK
  Top 0.254: IC1.21 50.99,24.32
  Top 0.406: 50.99,24.32 49.53,22.86 49.53,13.97 46.99,11.43 X2.2
SWDIO
  Top 0.254: 48.26,22.86 50.49,25.09 IC1.20
  Top 0.406: 48.26,22.86 48.26,16.51 X2.1
TS_PWM/SDA
  Top 0.254: JP2.3 74.3,14.61 65.41,14.61 60.96,19.05 60.96,32.89 56.52,37.34 56.52,38.73 55.92,39.33 IC1.43
TS_SCL
  Top 0.254: JP2.4 66.04,12.7 60.33,18.41 60.33,32.64 55.88,37.08 55.88,38.61 55.66,38.83 IC1.42
VCCD  (via drill 0.6)
  Top 0.254: IC1.86 38.37,37.83 38.1,38.1 37.47,38.73 36.83,39.37 v36.83,40.64 | IC1.39 53.48,37.33 v52.07,38.73
  Top 0.406: C25.1 37.47,38.73
  Bottom 0.254: v36.83,40.64 38.73,38.73 v52.07,38.73 53.72,37.08 C24.1
VIN_MON
  Top 0.254: 34.9,22.99 IC1.1
  Top 0.406: R35.2 C32.1 | C32.1 25.66,25.27 R34.1 | C32.1 34.9,22.99

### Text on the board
_tsilk: CONTRAST | UP | G1 | DN | G2 | L | G3 | R | G4 | MID | H2 | BT_RX | BT_TX | HC | H1 | TS | AR | MC | BT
